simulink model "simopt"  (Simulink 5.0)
settings: Solver=ode5  StartTime=0.0  StopTime=10  FixedStep=0.01  RelTol=1e-3

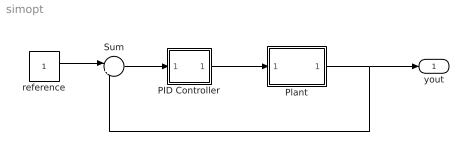
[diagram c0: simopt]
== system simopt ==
  PID Controller : Subsystem  mask(PID Controller){}
      mask help: Enter expressions for proportional, integral, and derivative terms. P+I/s+Ds
      mask init:
      | P=@1; I=@2; D=@3;
  Plant : Subsystem
  Sum : Sum  Inputs=|+-
  reference : Constant
  yout : Outport
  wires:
  Sum/1 -> PID Controller/1(In_1)
  Plant/1(y) -> Sum/2, yout/1
  reference/1 -> Sum/1
  PID Controller/1(Out_1) -> Plant/1(u)

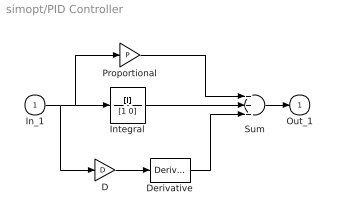
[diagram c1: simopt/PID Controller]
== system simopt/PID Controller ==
  In_1 : Inport
  D : Gain  Gain=D
  Derivative : Derivative
  Integral : TransferFcn  Numerator=[I]  Denominator=[1 0]
  Proportional : Gain  Gain=P
  Sum : Sum  Inputs=+++
  Out_1 : Outport  InitialOutput=0
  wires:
  Proportional/1 -> Sum/1
  Integral/1 -> Sum/2
  Derivative/1 -> Sum/3
  In_1/1 -> Integral/1, Proportional/1, D/1
  Sum/1 -> Out_1/1
  D/1 -> Derivative/1

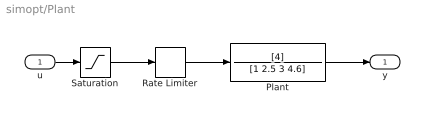
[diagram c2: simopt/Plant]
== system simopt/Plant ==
  u : Inport
  Plant : TransferFcn  Numerator=[4]  Denominator=[1 2.5 3 4.6]
  Rate Limiter : RateLimiter  RisingSlewLimit=3  FallingSlewLimit=-3
  Saturation : Saturate  UpperLimit=8  LowerLimit=-8
  y : Outport
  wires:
  Saturation/1 -> Rate Limiter/1
  Rate Limiter/1 -> Plant/1
  Plant/1 -> y/1
  u/1 -> Saturation/1
